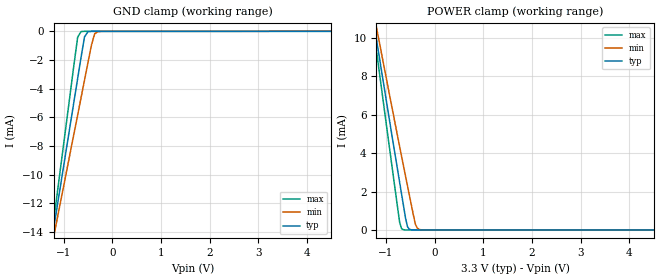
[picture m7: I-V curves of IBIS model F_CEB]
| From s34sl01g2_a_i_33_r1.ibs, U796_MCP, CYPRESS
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|   Model   F_CEB
[Model]   F_CEB
Model_type Input
Vinl =   0.6600V
Vinh =   2.6400V
   C_comp   1.4223pF   1.4145pF   1.4260pF
[Temperature Range]   25.0000   0.1050k   -40.0000
[Pullup Reference]   3.3000V   3.0000V   3.6000V
[Pulldown Reference]   0.0V   0.0V   0.0V
[POWER Clamp Reference]   3.3000V   3.0000V   3.6000V
[GND Clamp Reference]   0.0V   0.0V   0.0V
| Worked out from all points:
|   GND clamp passes 1 mA (typ) near -0.60 V on its own axis
|   POWER clamp passes 1 mA (typ) near -0.62 V on its own axis
[GND_clamp]
|Voltage   I(typ)   I(min)   I(max)
-3.3V     -58.25mA   -50.51mA   -68.01mA
-1.27V    -15.17mA   -15.49mA   -14.97mA
-1.2V     -13.69mA   -14.29mA   -13.14mA
-1.13V    -12.2mA    -13.08mA   -11.31mA
-710mV    -3.287mA   -5.833mA   -407.1uA
-640mV    -1.802mA   -4.625mA   -14.79uA
-570mV    -392.7uA   -3.418mA   -1.334uA
-500mV    -28.41uA   -2.21mA    -916.6nA
-430mV    -2.329uA   -1.003mA   -902.8nA
-360mV    -604.8nA   -162.9uA   -902.3nA
-290mV    -490.1nA   -19.76uA   -902.2nA
6.6V      39.72pA    16.99uA    -233.3nA
[POWER_clamp]
|Voltage   I(typ)   I(min)   I(max)
-3.28V    42.98mA    38.08mA    49.06mA
-1.28V    11.24mA    11.65mA    10.92mA
-1.24V    10.61mA    11.12mA    10.16mA
-1.2V     9.976mA    10.6mA     9.399mA
-1.16V    9.344mA    10.07mA    8.639mA
-720mV    2.468mA    4.337mA    379.5uA
-680mV    1.854mA    3.828mA    64.23uA
-640mV    1.24mA     3.32mA     9.947uA
-560mV    171.1uA    2.309mA    809.7nA
-400mV    603.9nA    322.6uA    371.8nA
-280mV    161.8nA    9.267uA    251.9nA
6.6V      39.72pA    2.996nA    43.19pA
